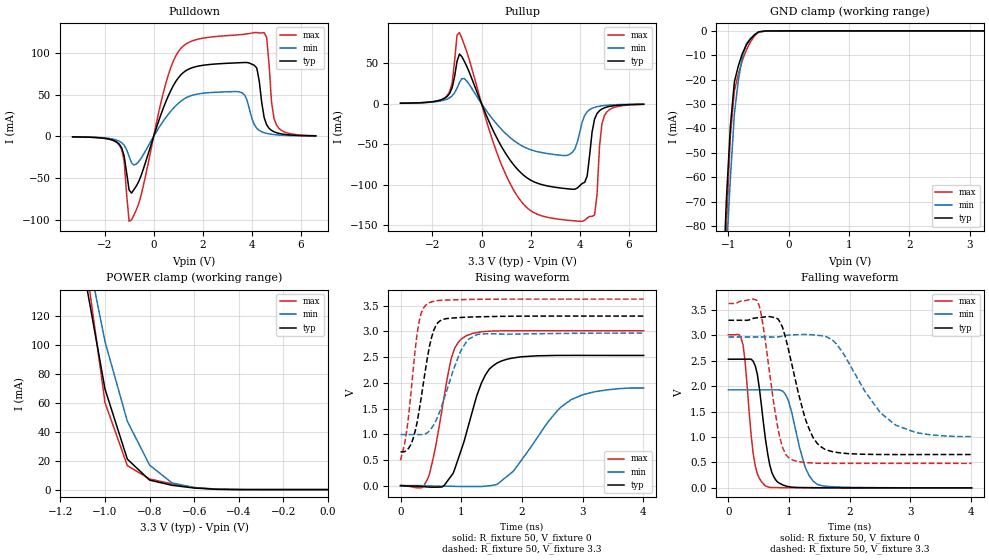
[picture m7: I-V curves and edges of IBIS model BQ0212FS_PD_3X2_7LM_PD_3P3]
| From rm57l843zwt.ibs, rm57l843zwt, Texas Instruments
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|   Model Cell FS_PD_3X2_7LM_PD_3P3
|BQ0212FS_PD_3X2_7LM_PD_3P3
[Model]   BQ0212FS_PD_3X2_7LM_PD_3P3
Model_type   I/O
Polarity   Non-Inverting
Enable   Active-Low
Vinl =  1.25
Vinh =  1.65
Cref =  15.0001pF
Rref =  101.0000M
Vref =  0V
Vmeas =  1.65
C_comp   1.2p   1.2p   1.2p
[Model Spec]
Vinl   1.25   1.12   1.38
Vinh   1.65   1.45   1.75
[Temperature Range]   25   155   -40
[Voltage Range]   3.3   2.97   3.63
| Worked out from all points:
|   slope of the pulldown table from 0 to 0.495 V, typ, clamps not added: 11.9 ohm
|   slope of the pullup table from 0 to 0.495 V, typ, clamps not added: 14.3 ohm
|   GND clamp passes 1 mA (typ) near -0.53 V on its own axis
|   POWER clamp passes 1 mA (typ) near -0.59 V on its own axis
|   rising waveform, R_fixture 50, V_fixture 0: 20-80 % time 400ps typ, 715ps min, 275ps max; typ from 0 V to 2.53 V
|   rising waveform, R_fixture 50, V_fixture 3.3: 20-80 % time 224ps typ, 347ps min, 172ps max; typ from 0.656 V to 3.3 V
|   falling waveform, R_fixture 50, V_fixture 0: 20-80 % time 171ps typ, 243ps min, 139ps max; typ from 2.53 V to 0 V
|   falling waveform, R_fixture 50, V_fixture 3.3: 20-80 % time 342ps typ, 655ps min, 230ps max; typ from 3.3 V to 0.656 V
[POWER_clamp]
|   voltage   I(typ)   I(min)   I(max)
-3.3V     2.375A     2.63A      3.153A
-1.1V     156mA      180.2mA    173.4mA
-1.067V   127.2mA    154.3mA    135.7mA
-1.033V   98.42mA    128.4mA    97.94mA
-1V       69.62mA    102.5mA    60.22mA
-900mV    21.14mA    47.42mA    16.64mA
-800mV    6.593mA    17.01mA    7.345mA
-700mV    3.017mA    4.694mA    4.027mA
-600mV    1.106mA    1.412mA    1.463mA
-500mV    206.7uA    366.5uA    241.6uA
0V        19.75uA    8.57uA     38.26uA
[Pulldown]
|   voltage   I(typ)   I(min)   I(max)
-3.3V     -554.3uA   -511.5uA   -526.2uA
-1.4V     -9.291mA   -5.703mA   -10.34mA
-1.2V     -23.68mA   -10.64mA   -30.19mA
-1V       -64.35mA   -24mA      -101.9mA
-600mV    -53.61mA   -29.92mA   -79.98mA
1V        70.16mA    39.6mA     101.5mA
3.5V      88.44mA    53.42mA    122.1mA
4.2V      81.93mA    9.711mA    124.7mA
4.6V      13.96mA    3.646mA    118.8mA
4.8V      7.183mA    2.57mA     41.14mA
5V        4.453mA    1.905mA    13.75mA
6.6V      621.1uA    479.2uA    840.9uA
[Pullup]
|   voltage   I(typ)   I(min)   I(max)
-3.3V     614.6uA    591.9uA    551.1uA
-1.4V     9.028mA    5.738mA    10.01mA
-900mV    61.32mA    26.24mA    87.8mA
1.4V      -78.76mA   -47.33mA   -111.2mA
3.5V      -105mA     -63.56mA   -143.7mA
4.1V      -98.29mA   -22.39mA   -145.1mA
4.3V      -89.13mA   -9.839mA   -141.1mA
4.6V      -19.02mA   -4.469mA   -137.2mA
4.7V      -12.15mA   -3.653mA   -112.5mA
4.8V      -8.616mA   -3.042mA   -53.65mA
5V        -5.089mA   -2.205mA   -14.76mA
6.6V      -663.5uA   -536.5uA   -825.6uA
[GND_clamp]
|   voltage   I(typ)   I(min)   I(max)
-3.3V     -1.947A    -1.623A    -3.254A
-1.1V     -112mA     -127mA     -135.8mA
-1.033V   -69.61mA   -91.63mA   -80.19mA
-966.7mV  -39.23mA   -60.62mA   -43.12mA
-900mV    -20.87mA   -34.02mA   -24.53mA
-833.3mV  -14.26mA   -20.12mA   -17.62mA
-766.7mV  -9.202mA   -10.52mA   -12.02mA
-700mV    -5.679mA   -5.211mA   -7.726mA
-566.7mV  -1.577mA   -1.578mA   -2.073mA
-500mV    -412.7uA   -590.8uA   -476.8uA
-300mV    -6.976uA   -10.31uA   -10.43uA
3.233V    19.75uA    12.57uA    38.26uA
[Ramp]
| variable   typ   min   max
dV/dt_f   1.631628/0.3489526n   1.217183/0.6769872n   1.941531/0.2340601n
dV/dt_r   1.539856/0.4017589n   1.169988/0.7436984n   1.835313/0.2782155n
R_load = 50
[Rising Waveform]
R_fixture = 50
V_fixture = 0
V_fixture_min = 0
V_fixture_max = 0
|   time   V(typ)   V(min)   V(max)
0s        299.8uV    -1.156uV   -9.816mV
340ps     -15.61mV   -291uV     -44.71mV
444ps     -27.3mV    -6.957mV   122.3mV
580ps     -31.73mV   -9.746mV   766.1mV
840ps     195mV      -13.94mV   2.488V
1.072ns   965.1mV    -18.18mV   2.91V
1.332ns   1.991V     -18.31mV   2.993V
1.66ns    2.424V     88.11mV    3.013V
2.812ns   2.534V     1.673V     3.014V
4.008ns   2.533V     1.899V     3.014V
[Rising Waveform]
R_fixture = 50
V_fixture = 3.3
V_fixture_min = 2.97
V_fixture_max = 3.63
|   time   V(typ)   V(min)   V(max)
0s        656.2mV    993.3mV    492.6mV
104ps     687.8mV    993.3mV    1.078V
204ps     900.7mV    993.4mV    2.199V
308ps     1.469V     991.9mV    3.203V
444ps     2.496V     1.03V      3.541V
544ps     3.015V     1.174V     3.588V
648ps     3.205V     1.444V     3.605V
996ps     3.273V     2.63V      3.619V
1.256ns   3.285V     2.937V     3.627V
4.008ns   3.3V       2.969V     3.63V
[Falling Waveform]
R_fixture = 50
V_fixture = 0
V_fixture_min = 0
V_fixture_max = 0
|   time   V(typ)   V(min)   V(max)
0s        2.533V     1.929V     3.014V
240ps     2.533V     1.929V     2.817V
408ps     2.493V     1.929V     675mV
476ps     2.238V     1.929V     279.3mV
612ps     941.4mV    1.929V     34.91mV
716ps     300.6mV    1.929V     7.554mV
944ps     37.47mV    1.828V     3.415mV
1.256ns   5.637mV    440.4mV    1.094mV
1.464ns   3.232mV    68.88mV    672.9uV
4.008ns   99.11uV    796.3uV    -2.303uV
[Falling Waveform]
R_fixture = 50
V_fixture = 3.3
V_fixture_min = 2.97
V_fixture_max = 3.63
|   time   V(typ)   V(min)   V(max)
0s        3.3V       2.97V      3.63V
476ps     3.349V     2.97V      3.684V
580ps     3.362V     2.97V      3.13V
816ps     3.326V     2.972V     1.166V
892ps     3.161V     2.99V      793.3mV
1.024ns   2.542V     3.01V      567.7mV
1.28ns    1.314V     3.02V      497.1mV
1.592ns   757mV      2.989V     483.3mV
2.756ns   655.7mV    1.235V     482.4mV
4.008ns   656.5mV    1.01V      482.1mV
